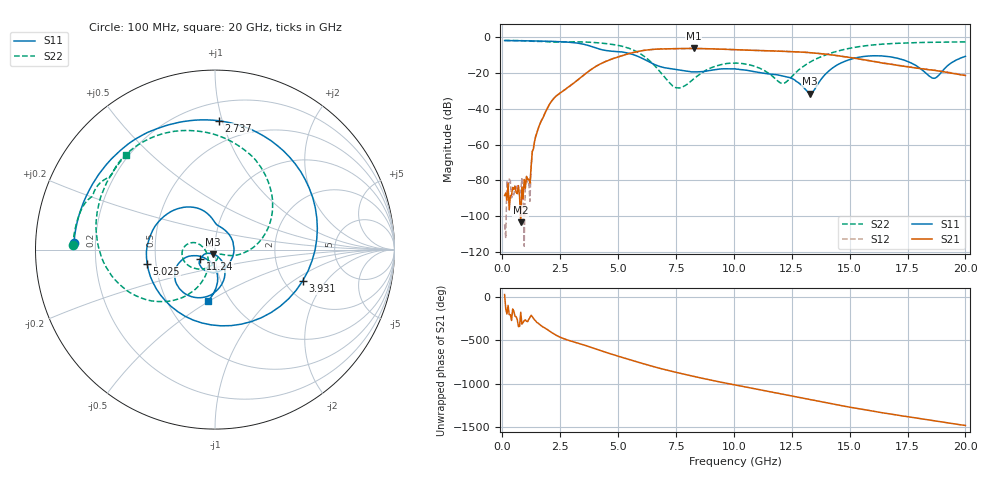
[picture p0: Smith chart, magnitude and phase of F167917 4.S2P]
!  2-Port S-parameters saved by WinCal
! VAR MeasName=S-Parameters (CALIBRATED_DATA) read from VNA (N5242A)
! VAR MeasDate=2016-11-22 8:59:50
! VAR NAME=F167917 4
! VAR FILENAME=F167917 4.S2P
! VAR DATE=2016-11-22 8:59:50
! VAR PHYS_PORTS=1,2
# Hz S DB R 50
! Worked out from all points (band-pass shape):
!   401 points, 100 MHz to 20 GHz, reference 50 ohm
!   highest |S21| = -6.47 dB at 8.259 GHz (marker M1); lowest = -103.4 dB at 796.5 MHz (marker M2)
!   |S21| within 3 dB of the highest: 5.433 GHz to 13.82 GHz (8.387 GHz wide, 87.1 % of centre)
!   lowest |S11| = -31.6 dB at 13.28 GHz (marker M3), VSWR 1.05, Z = 49 - j2.39 ohm
!   |S11| at or under -10 dB: 5.676 GHz to end of sweep
!   |S22| runs from -28.5 to -2.0 dB; largest |S21 - S12| = 0.0045
!   S11 on the Smith chart (normalised r, x): 100 MHz: 0.12, +0.02; 2.737 GHz: 0.33, +0.97; 3.931 GHz: 2.49, -1.20; 5.025 GHz: 0.45, -0.08; 11.24 GHz: 0.84, -0.09; 20 GHz: 0.79, -0.49
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1e8  -2.09 177.3  -88.44 27.8  -104.50 -41.5  -2.03 178.3
7.965e8  -2.19 158.8  -103.37 -176.2  -85.47 -122.4  -2.13 166.5
1.14475e9  -2.25 149.1  -79.30 103.5  -81.78 104.0  -2.29 160.3
1.493e9  -2.30 138.7  -53.44 66.5  -53.65 66.7  -2.55 155.6
1.94075e9  -2.43 123.5  -39.87 -14.3  -39.82 -14.8  -2.72 148.0
2.73675e9  -2.87 88.4  -29.18 -127.7  -29.18 -128.1  -2.81 137.1
3.43325e9  -3.93 37.7  -22.19 175.4  -22.21 175.2  -2.86 122.0
3.93075e9  -5.71 -19.8  -17.38 131.9  -17.37 132.1  -3.14 108.9
4.3785e9  -7.41 -85.4  -14.24 91.0  -14.18 90.9  -3.63 95.5
5.02525e9  -8.27 -168.1  -11.13 36.5  -11.09 36.0  -4.83 72.1
6.7665e9  -16.37 90.3  -6.79 -98.4  -6.82 -98.5  -18.76 -16.2
7.51275e9  -18.26 64.1  -6.57 -147.6  -6.60 -147.7  -28.36 -40.6
8.259e9  -19.52 5.9  -6.47 166.8  -6.49 167.0  -23.49 -87.8
1.005e10  -17.86 -122.6  -7.15 67.2  -7.15 67.4  -14.65 -169.0
1.1244e10  -20.16 -147.6  -7.70 6.5  -7.68 6.5  -18.27 161.5
1.21395e10  -21.86 -152.5  -8.08 -39.1  -8.05 -39.2  -25.90 -154.2
1.328375e10  -31.60 -112.2  -8.83 -99.0  -8.84 -98.9  -14.14 -112.4
1.338325e10  -31.07 -92.0  -8.92 -104.4  -8.94 -104.1  -13.42 -113.5
1.467675e10  -14.29 -78.1  -10.85 -171.4  -10.82 -171.1  -7.31 -137.9
1.67165e10  -11.08 -142.5  -15.15 95.3  -15.12 95.5  -3.84 -179.2
1.865675e10  -23.10 -121.3  -18.65 15.7  -18.59 15.8  -3.03 150.8
2e10  -10.87 -97.4  -21.54 -38.1  -21.32 -38.0  -2.84 133.4
